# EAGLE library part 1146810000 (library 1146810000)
PCB plug-in connector, male header, open side, THT solder connection, 5.08 mm, Number of poles: 6, 90, Solder pin length: 3.2 mm, tinned, orange, Box Source: Datasheet
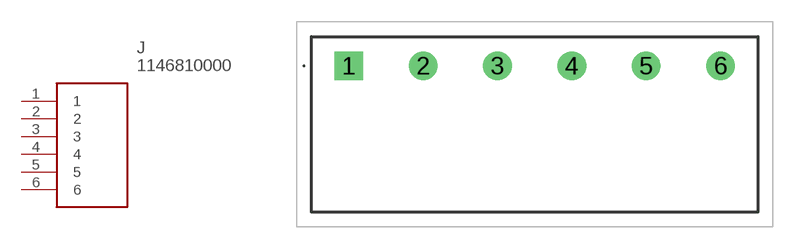
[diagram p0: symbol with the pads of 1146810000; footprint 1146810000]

Designator prefix J

## 1146810000 (Description: PCB plug-in connector, male header, open side, THT solder connection, 5.08 mm, Number of poles: 6, 90, Solder pin length: 3.2 mm, tinned, orange, Box; Height: 8.4mm; Manufacturer_Name: Weidmuller; Manufacturer_Part_Number: 1146810000)  [1146810000]
1  1
2  2
3  3
4  4
5  5
6  6

## Footprint 1146810000 (pad centres in mm)
1146810000-2
drill 1.3 pad 1.95 square: 1 0,0
drill 1.3 pad 1.95: 2 5.08,0; 3 10.16,0; 4 15.24,0; 5 20.32,0; 6 25.4,0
